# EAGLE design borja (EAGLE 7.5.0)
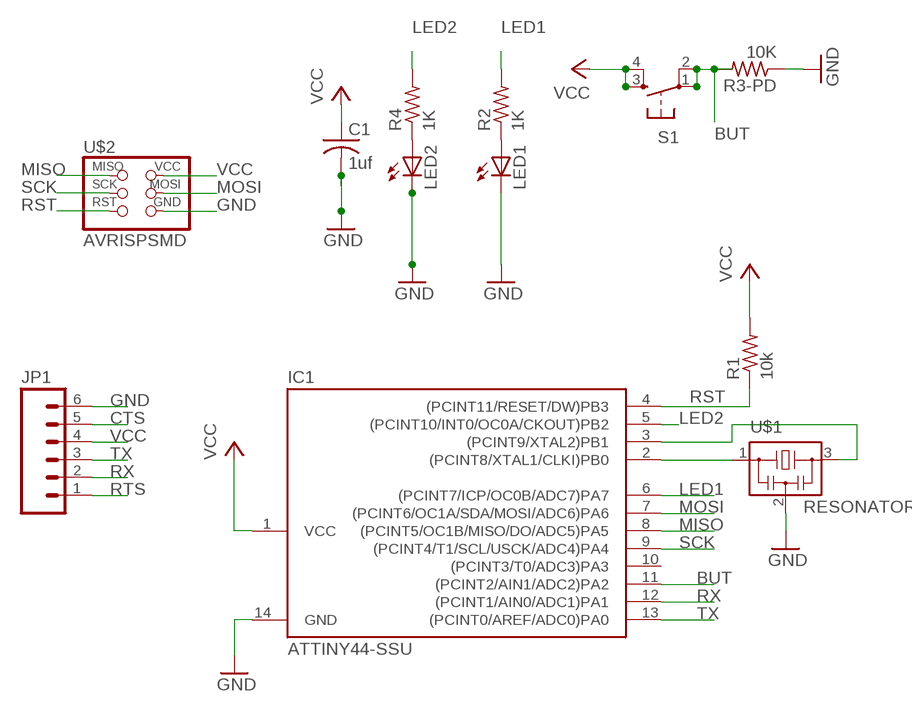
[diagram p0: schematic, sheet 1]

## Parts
C1  1uf  C-USC1206  [C1206]
IC1  ATTINY44-SSU  [SOIC14]
JP1  M06SMD  [1X06-SMD]
LED1  LEDFAB1206  [LED1206FAB]
LED2  LEDFAB1206  [LED1206FAB]
R1  10k  R-US_R1206  [R1206]
R2  1K  RES-US1206FAB  [R1206FAB]
R3-PD  10K  RES-US1206FAB  [R1206FAB]
R4  1K  RES-US1206FAB  [R1206FAB]
S1  6MM_SWITCH6MM_SWITCH  [6MM_SWITCH]
U$1  RESONATOR  [EFOBM]
U$2  AVRISPSMD  [2X03SMD]

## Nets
BUT: IC1.11((PCINT2/AIN1/ADC2)PA2) R3-PD.2 S1.1(P) S1.2(P1)
CTS: JP1.5
GND: C1.2 IC1.14(GND) JP1.6 LED1.2(C) LED2.2(C) R3-PD.1 U$1.2 U$2.6(GND)
LED1: IC1.6((PCINT7/ICP/OC0B/ADC7)PA7) R2.2
LED2: IC1.5((PCINT10/INT0/OC0A/CKOUT)PB2) R4.2
MISO: IC1.8((PCINT5/OC1B/MISO/DO/ADC5)PA5) U$2.1(MISO)
MOSI: IC1.7((PCINT6/OC1A/SDA/MOSI/ADC6)PA6) U$2.4(MOSI)
N$1: IC1.2((PCINT8/XTAL1/CLKI)PB0) U$1.1
N$2: IC1.3((PCINT9/XTAL2)PB1) U$1.3
N$3: LED1.1(A) R2.1
N$4: LED2.1(A) R4.1
RST: IC1.4((PCINT11/RESET/DW)PB3) R1.1 U$2.5(RST)
RTS: JP1.1
RX: IC1.12((PCINT1/AIN0/ADC1)PA1) JP1.2
SCK: IC1.9((PCINT4/T1/SCL/USCK/ADC4)PA4) U$2.3(SCK)
TX: IC1.13((PCINT0/AREF/ADC0)PA0) JP1.3
VCC: C1.1 IC1.1(VCC) JP1.4 R1.2 S1.3(S) S1.4(S1) U$2.2(VCC)
Unconnected: IC1.10((PCINT3/T0/ADC3)PA3)

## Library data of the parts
C1 = rcl:C-US: CAPACITOR, American symbol
IC1 = fab:ATTINY44
JP1 = SparkFun:M06: Header 6 Standard 6-pin 0.1" header. Use with straight break away headers (SKU : PRT-00116), right angle break away headers (PRT-00553), swiss pins (PRT-00743), machine pins (PRT-00117), and female headers (PRT-00115). Molex polarized connector foot print use with SKU : PRT-08094 with associated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
LED1 LED2 = 01fab:LED: LED
R1 = resistor:R-US_: RESISTOR, American symbol
R2 R3-PD R4 = 01fab:RES-US: Resistor (US Symbol)
S1 = 01fab:6MM_SWITCH: OMRON SWITCH
U$1 = fab:RESONATOR
U$2 = fab:AVRISP

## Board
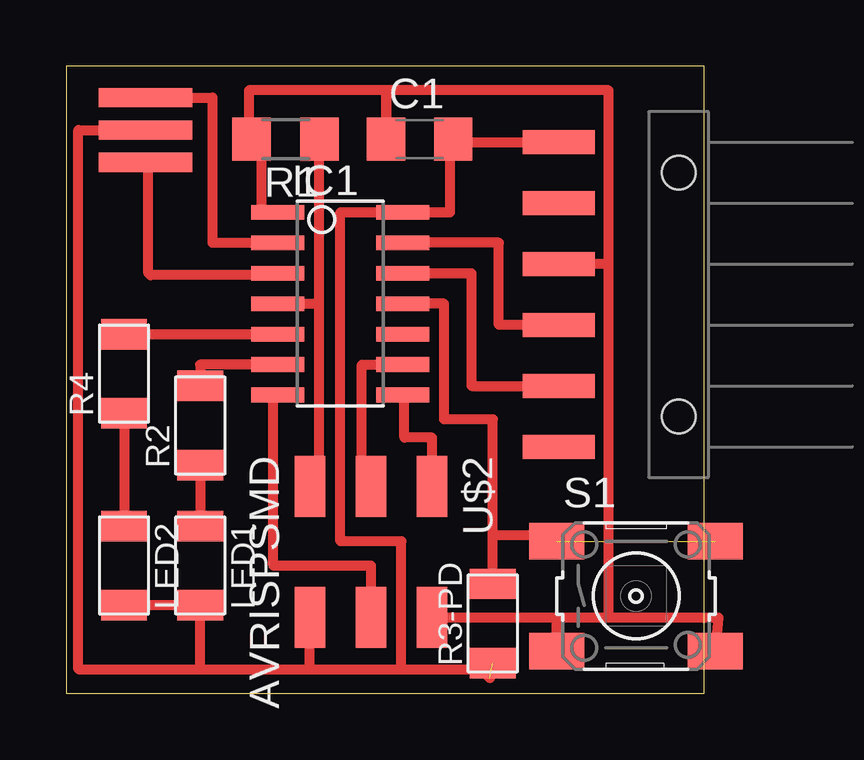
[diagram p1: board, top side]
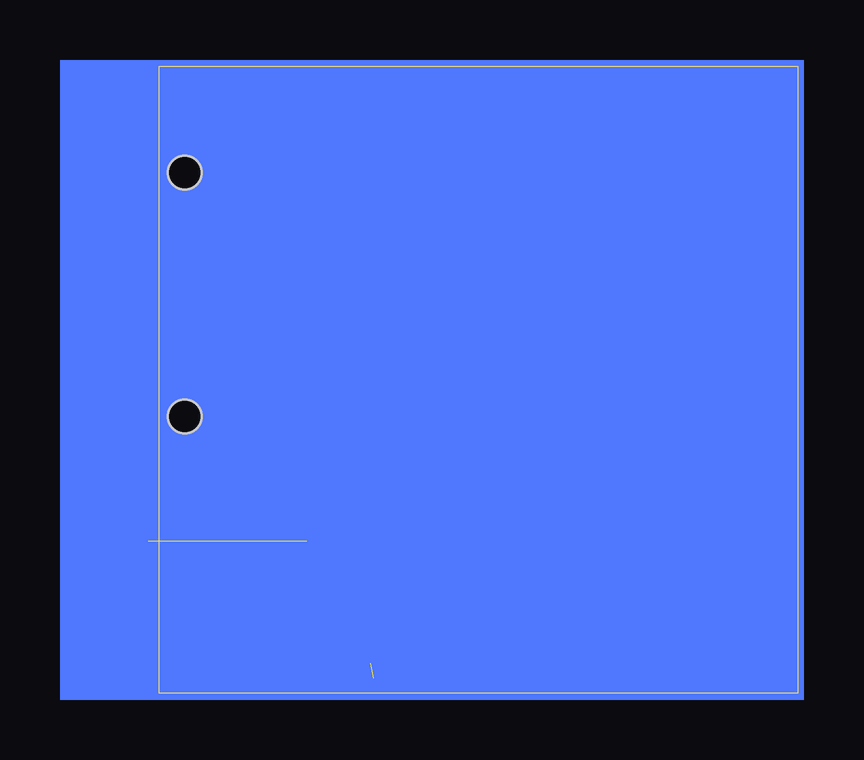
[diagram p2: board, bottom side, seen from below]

Size 26.59 x 26.15 mm. Coordinates in mm from the lower left corner, seen from the top.
Outline: 0,0 26.59,0 26.59,26.15 0,26.15 0,0
Copper layers 1: Top 0.035mm
Design rules "ERP-1sided-10mil-16mill *": minimum track width 18mil, minimum drill 32mil, track to track 0.41mm, track to pad 0.41mm, pad to pad 0.41mm, via to via 0.41mm, smd to smd 0.41mm, copper to edge 1mil, drill to drill 8mil, minimum pad ring 10mil, minimum via ring 8mil, stop-mask expansion 4mil, vias tented up to drill 0mil, thermal gap 10mil

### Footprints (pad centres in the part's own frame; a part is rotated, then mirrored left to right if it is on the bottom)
C1206 = smd 1.6 x 1.8: 1 -1.4,0; 2 1.4,0
SOIC14 = smd 0.61 x 2.21: 1 -3.81,-2.603; 2 -2.54,-2.603; 3 -1.27,-2.603; 4 0,-2.603; 5 1.27,-2.603; 6 2.54,-2.603; 7 3.81,-2.603; 8 3.81,2.603; 9 2.54,2.603; 10 1.27,2.603; 11 0,2.603; 12 -1.27,2.603; 13 -2.54,2.603; 14 -3.81,2.603
1X06-SMD = smd 1 x 3: 1 -6.35,5; 2 -3.81,5; 3 -1.27,5; 4 1.27,5; 5 3.81,5; 6 6.35,5 | hole 1.4: -5.08,0; 5.08,0
LED1206FAB = smd 1.27 x 1.905: 1 -1.651,0; 2 1.651,0
R1206 = smd 1.6 x 1.803: 1 -1.422,0; 2 1.422,0
R1206FAB = smd 1.27 x 1.905: 1 -1.651,0; 2 1.651,0
6MM_SWITCH = smd 2.286 x 1.524: 1 -3.302,2.286; 2 3.302,2.286; 3 -3.302,-2.286; 4 3.302,-2.286
EFOBM = smd 0.8 x 3.9: 1 -1.35,0; 2 0,0; 3 1.35,0
2X03SMD = smd 2.54 x 1.27: 1 -2.54,2.54; 2 2.92,2.54; 3 -2.54,0; 4 2.92,0; 5 -2.54,-2.54; 6 2.92,-2.54

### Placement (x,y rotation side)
C1  14.73,23.11 0 top
IC1  11.43,16.26 270 top
JP1  25.53,16.64 90 top
LED1  5.59,5.33 270 top
LED2  2.41,5.33 270 top
R1  9.14,23.11 180 top
R2  5.59,11.18 90 top
R3-PD  17.78,2.92 90 top
R4  2.41,13.34 90 top
S1  23.75,4.06 0 top
U$1  3.3,23.5 270 top
U$2  12.7,6.1 270 top

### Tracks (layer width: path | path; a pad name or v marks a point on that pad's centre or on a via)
BUT  (1 unrouted)
  Top 0.406: R3-PD.2 17.78,6.6 | 17.78,6.6 20.45,6.6 S1.1 | 17.78,6.6 17.78,11.43 15.75,11.43 15.75,16.26 IC1.11
GND  (1 unrouted)
  Top 0.406: 13.97,1.02 13.97,6.35 11.43,6.35 11.43,20.07 IC1.14 16,20.07 16,23.11 C1.2 16.13,22.99 JP1.6 20.15,23.24 | 10.16,1.02 13.97,1.02 | U$1.2 0.51,23.5 0.51,1.02 5.59,1.02 | U$2.6 10.16,1.02 | 5.59,1.02 10.16,1.02 | LED2.2 LED1.2 5.59,1.02 | 13.97,1.02 17.27,1.02 17.65,0.64
LED1
  Top 0.406: IC1.6 5.59,13.72 R2.2
LED2
  Top 0.406: R4.2 IC1.5
MISO
  Top 0.406: U$2.1 15.24,10.67 14.1,10.67 14.1,12.38 IC1.8
MOSI
  Top 0.406: IC1.7 8.64,12.45 8.64,5.33 12.7,5.33 U$2.4
N$1
  Top 0.406: U$1.1 6.1,24.84 6.1,18.8 IC1.2
N$2
  Top 0.406: 3.43,22.14 U$1.3 3.43,22.02 3.43,17.53 3.51,17.45 8.83,17.45 IC1.3
N$3
  Top 0.406: R2.1 LED1.1
N$4
  Top 0.406: R4.1 LED2.1
RST
  Top 0.406: R1.1 10.54,23.11 10.54,16.26 | IC1.4 10.54,16.26 | U$2.5 10.54,8.64 10.54,16.26
RX
  Top 0.406: IC1.12 16.89,17.53 16.89,12.83 JP1.2
SCK
  Top 0.406: U$2.3 12.32,8.64 12.32,13.72 IC1.9
TX
  Top 0.406: JP1.3 18.03,15.37 18.03,18.8 IC1.13
VCC
  Top 0.254: 22.61,4.32 22.61,4.42
  Top 0.406: 22.61,17.91 JP1.4 | 22.61,17.91 22.61,4.32 22.61,3.18 | IC1.1 8.13,20.07 8.13,23.11 R1.2 7.62,23.11 7.62,25.15 13.33,25.15 C1.1 13.34,25.15 22.61,25.15 22.61,17.91 | U$2.2 20.45,3.18 | 20.45,3.18 22.61,3.18 | S1.3 20.45,3.18 | 22.61,3.18 27.18,3.17 S1.4
(copper drawn outside any net)
  shapes: Bottom area x1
